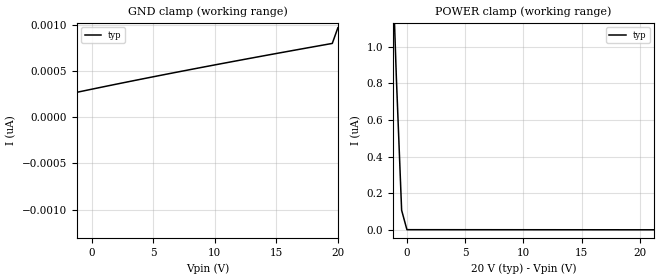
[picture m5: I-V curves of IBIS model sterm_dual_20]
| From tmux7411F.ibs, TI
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| sterm_dual_20
[Model]   sterm_dual_20
Model_type   Terminator
|   typ   min   max
C_comp   2.533030e-12   NA   NA
[Voltage Range]   20   NA   NA
[Temperature Range]   27   NA   NA
[Power Clamp Reference]   20   NA   NA
[GND Clamp Reference]   0   NA   NA
[GND Clamp]
|   Voltage   I(typ)   I(min)   I(max)
-25V      -18.27uA   NA         NA
-20.45V   -9.038uA   NA         NA
-19.55V   -233.1pA   NA         NA
-14.09V   -104.6pA   NA         NA
-2.727V   225.6pA    NA         NA
4.545V    424.1pA    NA         NA
19.55V    796.1pA    NA         NA
20V       965.1pA    NA         NA
[POWER Clamp]
|   Voltage   I(typ)   I(min)   I(max)
-5V       8.864uA    NA         NA
-1.364V   1.681uA    NA         NA
-909.1mV  835.5nA    NA         NA
-454.5mV  107nA      NA         NA
0V        965.1pA    NA         NA
40V       -743.3pA   NA         NA
